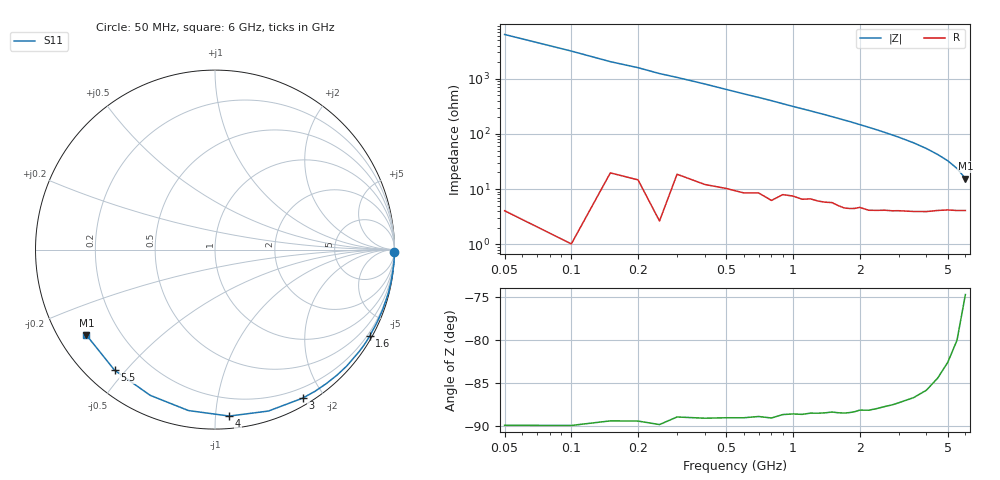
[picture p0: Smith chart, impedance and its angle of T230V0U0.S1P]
! SIEMENS Discrete & RF Semiconductors
! BAS70-04W
! Si Schottky Diode in SOT323
! VR = 30 V
! S-Parameters:  November  1997
# GHz  S  MA  R  50
!  f  S11
! GHz  MAG  ANG
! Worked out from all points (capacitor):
!   34 points, 50 MHz to 6 GHz, reference 50 ohm
!   read as one part to ground: C = 500 fF near 50 MHz
!   lowest |Z| = 15.6 ohm at 6 GHz (marker M1)
!   S11 on the Smith chart (normalised r, x): 50 MHz: open; 1.6 GHz: 0.10, -3.84; 3 GHz: 0.08, -1.75; 4 GHz: 0.08, -1.09; 5.5 GHz: 0.08, -0.47; 6 GHz: 0.08, -0.30
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0.05  1 -0.9
0.15  0.9995 -2.8
0.2  0.9994 -3.6
0.25  0.9998 -4.6
0.4  0.9981 -7.1
0.6  0.997 -10.7
0.7  0.996 -12.4
0.8  0.9962 -14.2
1  0.9927 -18.0
1.1  0.9923 -19.8
1.2  0.9907 -21.6
1.3  0.99 -23.5
1.4  0.9889 -25.3
1.6  0.9873 -29.2
1.7  0.9869 -31.2
1.8  0.9857 -33.1
1.9  0.9838 -35.2
2.2  0.9795 -41.5
2.4  0.9754 -45.8
2.6  0.9705 -50.3
2.8  0.9661 -54.9
3  0.9608 -59.5
3.5  0.9474 -71.7
4  0.9308 -85.1
4.5  0.9089 -99.4
5  0.8885 -114.0
5.5  0.8743 -129.8
6  0.8603 -146.4
